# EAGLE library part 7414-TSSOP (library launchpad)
Hex schmitt trigger INVERTER
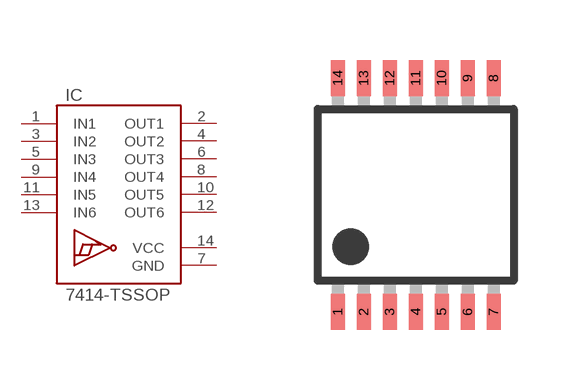
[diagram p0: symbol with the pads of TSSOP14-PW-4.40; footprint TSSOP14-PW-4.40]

Designator prefix IC

## 7414-TSSOP  [TSSOP14-PW-4.40]
1  IN1
2  OUT1
3  IN2
4  OUT2
5  IN3
6  OUT3
7  GND
8  OUT4
9  IN4
10  OUT5
11  IN5
12  OUT6
13  IN6
14  VCC

## Footprint TSSOP14-PW-4.40 (pad centres in mm)
plastic thin shrink small outline package; 14 leads; body width 4.4 mm SOT402-1 Source: http://www.nxp.com/documents/data_sheet/74ABT125.pdf
smd 0.35 x 0.9: 1 -1.95,-2.925; 2 -1.3,-2.925; 3 -0.65,-2.925; 4 0,-2.925; 5 0.65,-2.925; 6 1.3,-2.925; 7 1.95,-2.925; 8 1.95,2.925; 9 1.3,2.925; 10 0.65,2.925; 11 0,2.925; 12 -0.65,2.925; 13 -1.3,2.925; 14 -1.95,2.925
